PROGRAM MAIN
VAR
	bExecute				: BOOL;
	sLocalHost				: STRING(15);
	nLocalPort				: UDINT;
	asduAddr				: DWORD;
	nOrgAdd					: BYTE;
	hServer					: T_HSERVER; // TCP/IP server handle

	eComState				: E_ComState	:= INIT;
	fbConnection			: FB_ServerClientConnection;
	fbProtocol				: FB_IEC870_5_104TProtocol;
	stBuffer				: ST_IEC870_5_101TBuffer;
	fbBuffer				: FB_IEC870_5_101TBufferCtrl;
	
	stTxAsdu 				: ST_IEC870_5_101AOGen; // asdu to send 
	stRxAsdu 				: ST_IEC870_5_101AOGen; // received asdu 
	
	// general interrogation
	nQOI					: BYTE;
	
	// spontaneous data transmission
	fbSpontTime				: TON;
END_VAR

// timer
fbSpontTime(IN:= TRUE XOR fbSpontTime.Q, PT:= T#5S);

// connection management
CASE eComState OF
INIT: 
	// TCP/IP connection
	sLocalHost	:= '127.0.0.1';	// own (slave) ip-address
	nLocalPort	:= 2404;		// communication port - check firewall settings
	asduAddr	:= 3;			// common asdu address
	nOrgAdd		:= 1;
	
	// INIT protocol parameter
	fbConnection.eMode		:= eACCEPT_ALL;	// accept all incomming connections
	fbConnection.tReconnect	:= T#2S;

	fbProtocol.sSrvNetID				:= '';		
	fbProtocol.protPara.bPackFrames		:= TRUE;
	fbProtocol.protPara.bThrottleMode	:= TRUE;
	fbProtocol.bOutDbg					:= FALSE;	// disable debug output


	// INIT RX/TX buffer parameter
	stBuffer.eDbg		:= eIEC870_FIFO_DBG_ALL;
	stBuffer.asduFmt.eCOTSize		:= eIEC870_COT_TwoOctets;		// cause of transfer size
	stBuffer.asduFmt.eAsduAddrSize	:= eIEC870_AsduAddr_TwoOctets;	// common asdu addr size
	stBuffer.asduFmt.eObjAddrSize	:= eIEc870_ObjAddr_ThreeOctets;	// object address size

	eComState := IDLE;
		
		
IDLE:	
	IF bExecute THEN
		F_CreateServerHnd(	bEnable		:= FALSE,
							sSrvNetID	:= '',			// own (server) NetID
							sLocalHost	:= sLocalHost,
							nLocalPort	:= nLocalPort,
							nMode		:= LISTEN_MODE_CLOSeALL OR CONNECT_MODE_ENABLEDBG, // Close all previous opened and not closed sockets and enable debug messages on socket creation/connect/close
							hServer		:= hServer );	// create server connection handle
							
		stBuffer.asduSize := F_iecApdu104ToAsduLen(fbProtocol.protPara.APDULength);
		eComState := CONNECT;
	END_IF
	
		
CONNECT: 
	fbConnection( 	bEnable := bExecute,
					hServer	:= hServer );					
	CASE fbConnection.eState OF 
		eSOCKET_CONNECTED:
			fbProtocol.INIT( 	hSocket	:= fbConnection.hSocket, // reset fbProtocol and restart data transfer
								buffer	:= stBuffer );
			eComState := DATATRANSFER;			
		eSOCKET_DISCONNECTED:
			eComState := IDLE;	
		eSOCKET_SUSPENDED:
			; // wait for connection	
	END_CASE		
			
	
DATATRANSFER: 
	IF bExecute THEN
		fbProtocol(buffer := stBuffer);
		IF NOT fbProtocol.bError THEN
			IF fbProtocol.eDTState = eIEC870_STARTDT THEN	
				;// exchange data
			END_IF
		ELSE // error occured - log error msg. and close socket
			ADSLOGSTR(	ADSLOG_MSGTYPE_ERROR OR ADSLOG_MSGTYPE_LOG,		// log errors
						'IEC60870-5-104 Transport Interface error: %s',
						DWORD_TO_HEXSTR(fbProtocol.nErrID,0,TRUE));
			eComState := DISCONNECT;
		END_IF
	ELSE // stop data transfer
		eComState := DISCONNECT;
	END_IF
	
		
DISCONNECT: 
	fbProtocol(buffer := stBuffer);	
	fbConnection(	hServer := hServer,
					bEnable := FALSE );
					
	IF fbConnection.eState = eSOCKET_DISCONNECTED 
	AND fbProtocol.eDTState = eIEC870_STOPDT THEN
		eComState := IDLE;
	END_IF
END_CASE


// -----------------------------------------------------------------------------------
// process received data

REPEAT
	fbBuffer.RxRemoveObj(	getObj => stRxAsdu,
 							buffer := stBuffer);
								
	IF fbBuffer.bOk THEN
		CASE stRxAsdu.ident.eType OF
	
		C_IC_NA_1:	// interrogation command
			 
			F_iecCopyStreamToBuffer (ADR(nQOI),SIZEOF(nQOI), stRxAsdu.info.stream); //Copy value to local varialbe
			
					// create general interrogation confirmation asdu
					stTxAsdu := stRXAsdu;
					stTxAsdu.ident.eCOT := eIEC870_COT_ACT_CON; // cause of transfer -> activation confirmation
					fbBuffer.TxAddObj(	putObj := stTxAsdu,
										buffer := stBuffer);
					
					IF NOT fbBuffer.bOk THEN
						// code for buffer overflow
						EXIT; 
					END_IF
					
					// send general interrogation asdus - always without time tag
					
					// common stTxAsdu parameter 
					stTxAsdu.ident.asduAddr	:= asduAddr;
					stTxAsdu.ident.bSQ		:= FALSE;
					stTxAsdu.ident.nObj		:= 1;
					stTxAsdu.ident.eCOT		:= BYTE_TO_INT(nQOI);
					stTxAsdu.ident.nORG		:= stRxAsdu.ident.nORG;
					stTxAsdu.ident.bPN		:= FALSE;
					stTxAsdu.ident.bT		:= FALSE;
					stTxAsdu.ident.eClass	:= eIEC870_Class_1;
					
					
					// select datapoints to be sent in the respective groups
					IF (nQOI = eIEC870_QOI_INROGEN) THEN	// general interrogation
						// crete asdu (bSlaveToMaster)
						stTxAsdu.ident.eType	:= M_SP_NA_1;
						stTxAsdu.info.objAddr	:= 10;
						F_iecResetStream(0,stTxAsdu.info.stream);
						F_iecCopyBufferToStream(ADR(nSIQ_bSlaveToMaster),SIZEOF(nSIQ_bSlaveToMaster),stTxAsdu.info.stream);	// copy values TO transmit stream	
						fbBuffer.TxAddObj(	putObj:= stTxAsdu,
											buffer:= stBuffer);
						IF NOT fbBuffer.bOk THEN
							// code for buffer overflow
							EXIT; 
						END_IF			
					
						// create asdu (nBitstring)
						stTxAsdu.ident.eType	:= M_BO_NA_1;
						stTxAsdu.info.objAddr	:= 11;		// object address
						
						F_iecResetStream(0,stTxAsdu.info.stream);
						F_iecCopyBufferToStream(ADR(nBitstring),SIZEOF(nBitstring),stTxAsdu.info.stream);	// copy values TO transmit stream
						F_iecCopyBufferToStream(ADR(nQDS_nBitstring),SIZEOF(nQDS_nBitstring),stTxAsdu.info.stream);
						fbBuffer.TxAddObj(	putObj := stTxAsdu,
											buffer := stBuffer);
						IF NOT fbBuffer.bOk THEN
							// code for buffer overflow
							RETURN; 
						END_IF	 
					END_IF
					
					IF 	(nQOI = eIEC870_QOI_INRO1) OR
						(nQOI = eIEC870_QOI_INROGEN)THEN	// interrogation group 1 or general interrogation
						// create asdu (nMeasurementValue)
						stTxAsdu.ident.eType	:= M_ME_NB_1;
						stTxAsdu.info.objAddr	:= 12;		// object address
						
						F_iecResetStream(0,stTxAsdu.info.stream);
						F_iecCopyBufferToStream(ADR(nMeasurementValue),SIZEOF(nMeasurementValue),stTxAsdu.info.stream);	// copy values TO transmit stream
						F_iecCopyBufferToStream(ADR(nQDS_nMeasurementValue),SIZEOF(nQDS_nMeasurementValue),stTxAsdu.info.stream);
						fbBuffer.TxAddObj(	putObj := stTxAsdu,
											buffer := stBuffer);
						IF NOT fbBuffer.bOk THEN
							// code for buffer overflow
							RETURN; 
						END_IF	 
						
						// create asdu (fMeasurementValue)
						stTxAsdu.ident.eType	:= M_ME_NC_1;
						stTxAsdu.info.objAddr	:= 13;		// object address
						
						F_iecResetStream(0,stTxAsdu.info.stream);
						F_iecCopyBufferToStream(ADR(fMeasurementValue),SIZEOF(fMeasurementValue),stTxAsdu.info.stream);	// copy values TO transmit stream
						F_iecCopyBufferToStream(ADR(nQDS_fMeasurementValue),SIZEOF(nQDS_fMeasurementValue),stTxAsdu.info.stream);
						fbBuffer.TxAddObj(	putObj := stTxAsdu,
											buffer := stBuffer);
						IF NOT fbBuffer.bOk THEN
							// code for buffer overflow
							RETURN; 
						END_IF	
					END_IF
	
					// create interrogation activation termination asdu
					stTxAsdu := stRxAsdu;
					stTxAsdu.ident.eCOT := eIEC870_COT_ACT_TERM;	// cause of transfer -> activation termination
					fbBuffer.TxAddObj(	putObj:= stTxAsdu,
										buffer:= stBuffer);
					IF NOT fbBuffer.bOk THEN
						// code for buffer overflow
						EXIT; 
					END_IF		

				
		C_SC_NA_1: // single command without time tag
			CASE stRxAsdu.info.objAddr OF
			101:
				F_iecCopyStreamToBuffer(ADR(nSCO_bMasterToSlave),SIZEOF(nSCO_bMasterToSlave),stRxAsdu.info.stream);
				
				bMasterToSlave		:= nSCO_bMasterToSlave.0;
				eSCS_bMasterToSlave	:= BOOL_TO_INT(nSCO_bMasterToSlave.0);
				eQU_bMasterToSlave 	:= SHR((nSCO_bMasterToSlave AND 2#0111_1100),2);
				
				IF nSCO_bMasterToSlave.7 THEN
					; // code for select bit
				END_IF
			
				// create activation confirmation asdu
				stTxAsdu := stRxAsdu;
				stTxAsdu.ident.eCOT := eIEC870_COT_ACT_CON; //cause of transfer -> activation confirmation
				fbBuffer.TxAddObj(	putObj := stTxAsdu,
									buffer := stBuffer);
				IF NOT fbBuffer.bOk THEN
					// code for buffer overflow
					EXIT; 
				END_IF
				
				IF NOT nSCO_bMasterToSlave.7 THEN
					
					// code for execute function
					
					//create command activation termination asdu
					stTxAsdu := stRxAsdu;
					stTxAsdu.ident.eCOT := eIEC870_COT_ACT_TERM; // cause of transfer -> activation termination
					fbBuffer.TxAddObj(	putObj := stTxAsdu,
										buffer := stBuffer);
					IF NOT fbBuffer.bOk THEN
						// code for buffer overflow
						EXIT; 
					END_IF				
				END_IF
				
			ELSE 
				// code for invalid object address
				EXIT;  
			END_CASE
				
			// other asdu types
				
		ELSE
			// code for invalid asdu types
			EXIT;
		END_CASE
	END_IF

UNTIL NOT fbBuffer.bOk // RX fifo is empty
END_REPEAT


// -----------------------------------------------------------------------------------
// send data

IF fbSpontTime.Q THEN
	
	// bSlaveToMaster value manipulation - example
	bSlaveToMaster := NOT bSlaveToMaster;
	
	
	// bSlaveToMaster
	nSIQ_bSlaveToMaster.0	:= bSlaveToMaster;
	eSPI_bSlaveToMaster		:= BOOL_TO_INT(nSIQ_bSlaveToMaster.0);
	nSIQ_bSlaveToMaster		:= nSIQ_bSlaveToMaster OR SHL(INT_TO_BYTE(nQDS_bSlaveToMaster),4);
	nSIQ_bSlaveToMaster.7	:= 0;
	
	// common stTxAsdu parameter
	stTxAsdu.ident.asduAddr	:= asduAddr;		// common ASDU address
	stTxAsdu.ident.bSQ		:= FALSE;			// sequence - always false
	stTxAsdu.ident.nObj		:= 1;				// number of objects
	stTxAsdu.ident.eCOT		:= eIEC870_COT_SPONTAN;	// cause of transmission - spontaneous
	stTxAsdu.ident.nORG		:= nOrgAdd;			// originator address
	stTxAsdu.ident.bPN		:= FALSE;			// positive/ negative confirmation flag
	stTxAsdu.ident.bT		:= FALSE;			// test flag - not used
	stTxAsdu.ident.eClass	:= eIEC870_Class_1;	// priority class
	
	// create first asdu (bSlaveToMaster)
	stTxAsdu.ident.eType	:= M_SP_NA_1;
	stTxAsdu.info.objAddr	:= 10;				// object address
	
	F_iecResetStream(0,stTxAsdu.info.stream);
	F_iecCopyBufferToStream(ADR(nSIQ_bSlaveToMaster),SIZEOF(nSIQ_bSlaveToMaster),stTxAsdu.info.stream);	// copy values TO transmit stream
	fbBuffer.TxAddObj(	putObj := stTxAsdu,
						buffer := stBuffer);
	IF NOT fbBuffer.bOk THEN
		// code for buffer overflow
		RETURN; 
	END_IF	 
END_IF

END_PROGRAM
